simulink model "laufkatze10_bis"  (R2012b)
settings: Solver=ode45  StartTime=0.0  StopTime=10.0  RelTol=1e-3
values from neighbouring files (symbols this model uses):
  dft = 1    [laufkatze_1.m]    (also in laufkatze_10.m = 0.1)
  F0 = 2000    [laufkatze_1.m]    (also in laufkatze_10.m)
  g = 9.89    [fuellstnd_1.m]    (also in fuellstnd_2.m; fuellstnd_21.m; fuellstnd_3.m; fuellstnd_31.m)
  mk = 100    [laufkatze_1.m]    (also in laufkatze_10.m; laufkatze_2.m; laufkatze_20.m)
  mL = 500    [laufkatze_1.m]    (also in laufkatze_10.m; laufkatze_2.m; laufkatze_20.m)
  mu = 0.01    [laufkatze_10.m]    (also in laufkatze_20.m; feder_masse_1.m = 0.05; feder_masse_13.m = 0.05; feder_masse_14.m = 0.05)
  Tfinal = 2000    [aktiv_tilger_1.m]    (also in aktiv_tilger_12.m = 1000; aktiv_tilger_2.m = 1000; aktiv_tilger_3.m = 1000,         dt = 0.01; aktiv_tilger_31.m = 1000,         dt = 0.01)

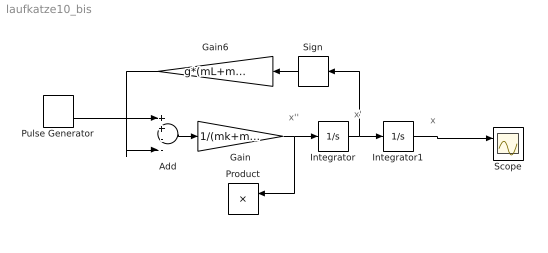
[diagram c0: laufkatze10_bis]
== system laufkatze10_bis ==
  note: x''
  note: x'
  note: x
  Add : Sum  Inputs=++--
  Gain : Gain  Gain=1/(mk+mL)
  Gain6 : Gain  Gain=g*(mL+mk)*mu
  Integrator : Integrator
  Integrator1 : Integrator
  Product : Product
  Pulse Generator : DiscretePulseGenerator  PulseType=Time based  Amplitude=F0  Period=Tfinal  PulseWidth=dft
  Scope : Scope  NumInputPorts=2
  Sign : Signum  ZeroCross=off
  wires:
  Pulse Generator/1 -> Add/1
  Add/1 -> Gain/1
  Gain/1 -> Integrator/1, Product/1
  Integrator/1 -> Integrator1/1, Sign/1
  ? -> Scope/2
  ? -> Product/2
  ? -> Add/3
  ? -> Add/2
  Product/1 -> ?
  Integrator1/1 -> Scope/1
  Sign/1 -> Gain6/1
  Gain6/1 -> Add/4
